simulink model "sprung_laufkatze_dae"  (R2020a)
settings: Solver=ode45  StartTime=0.0  StopTime=20  MaxStep=1e-2  RelTol=1e-5  EnableMultiTasking=on
libraries: simulink x1, simulink_extras x1

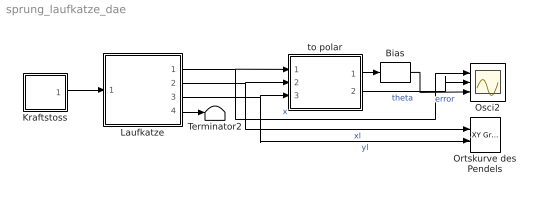
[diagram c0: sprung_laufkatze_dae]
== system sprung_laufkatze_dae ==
  Bias : Bias  Bias=-1
  Kraftstoss : Subsystem  mask(Kraftstoss){Ta=1, Te=10, A=100}
      mask prompts: Ta "Startzeit Te"; Te "Endzeit Ta"; A "Amplitude A"
      mask help: Rechtecksignal, das zur Zeit Te von 0 auf A geht, zur Zeit Ta dann wieder zurück auf 0.
  Laufkatze : Subsystem  mask(Laufkatze){mk=100, ml=1, L=1, g=9.81}
      mask prompts: mk "Laufkatzenmasse"; ml "Lastmasse"; L "Seillaenge"; g "Erdbeschleunigung"
      mask help: DAE-Modell einer Laufkatze als Regelstrecke
  Ortskurve des Pendels : simulink/Sinks/XY Graph  xmin=-1.2  xmax=140  ymin=-1.01  ymax=-0.95  st=-1
  Osci2 : Scope  NumInputPorts=3
  Terminator2 : Terminator
  to polar : Subsystem
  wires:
  Kraftstoss/1(Fext) -> Laufkatze/1(u)
  Laufkatze/1(x) -> to polar/1(x), Osci2/1  "x"
  Laufkatze/2(xl) -> to polar/2(xl), Ortskurve des Pendels/1  "xl"
  Laufkatze/3(yl) -> to polar/3(yl), Ortskurve des Pendels/2  "yl"
  to polar/1(l) -> Bias/1
  Bias/1 -> Osci2/3  "error"
  to polar/2(theta in Grad) -> Osci2/2  "theta"
  Laufkatze/4(lambda) -> Terminator2/1

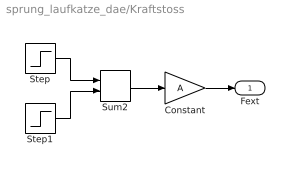
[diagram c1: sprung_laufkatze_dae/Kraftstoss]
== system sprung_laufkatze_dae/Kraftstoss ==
  Constant : Gain  Gain=A  SaturateOnIntegerOverflow=on
  Step : Step  Time=Ta  SampleTime=0
  Step1 : Step  Time=Te  After=-1  SampleTime=0
  Sum2 : Sum  InputSameDT=on  SaturateOnIntegerOverflow=on
  Fext : Outport
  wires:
  Constant/1 -> Fext/1
  Step1/1 -> Sum2/2
  Step/1 -> Sum2/1
  Sum2/1 -> Constant/1

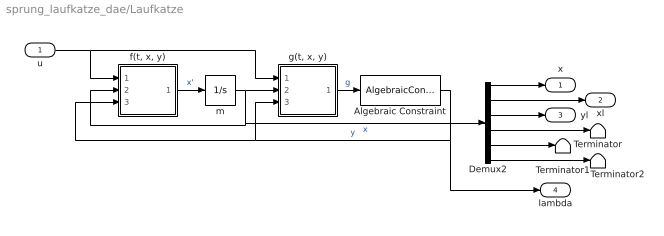
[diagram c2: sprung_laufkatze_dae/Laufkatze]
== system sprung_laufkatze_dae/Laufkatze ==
  u : Inport
  Algebraic Constraint : AlgebraicConstraint
  Demux2 : Demux  Outputs=6
  Terminator : Terminator
  Terminator1 : Terminator
  Terminator2 : Terminator
  "f(t, x, y)" : Subsystem
  "g(t, x, y)" : Subsystem
  m : Integrator  InitialCondition=[0,0,-L,0,0,0]'
  x : Outport
  xl : Outport  Port=2
  yl : Outport  Port=3
  lambda : Outport  Port=4
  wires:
  "g(t, x, y)"/1(g) -> Algebraic Constraint/1  "g"
  Algebraic Constraint/1 -> "g(t, x, y)"/3(y), "f(t, x, y)"/3(y), lambda/1  "y"
  m/1 -> "g(t, x, y)"/2(x), "f(t, x, y)"/2(x), Demux2/1  "x"
  "f(t, x, y)"/1(f) -> m/1  "x'"
  Demux2/1 -> x/1
  Demux2/2 -> xl/1
  Demux2/3 -> yl/1
  Demux2/4 -> Terminator/1
  Demux2/5 -> Terminator1/1
  Demux2/6 -> Terminator2/1
  u/1 -> "g(t, x, y)"/1(u), "f(t, x, y)"/1(u)

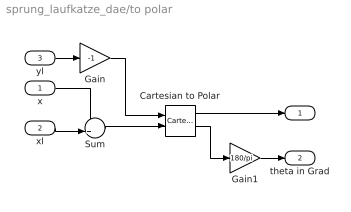
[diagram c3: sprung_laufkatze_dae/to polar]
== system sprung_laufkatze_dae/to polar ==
  x : Inport
  xl : Inport  Port=2
  yl : Inport  Port=3
  Cartesian to Polar : simulink_extras/Transformations/Cartesian to Polar
  Gain : Gain  Gain=-1
  Gain1 : Gain  Gain=180/pi
  Sum : Sum  Inputs=-+|
  l : Outport
  theta in Grad : Outport  Port=2
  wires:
  Cartesian to Polar/2 -> Gain1/1
  Cartesian to Polar/1 -> l/1
  x/1 -> Sum/1
  xl/1 -> Sum/2
  Sum/1 -> Cartesian to Polar/2
  yl/1 -> Gain/1
  Gain/1 -> Cartesian to Polar/1
  Gain1/1 -> theta in Grad/1

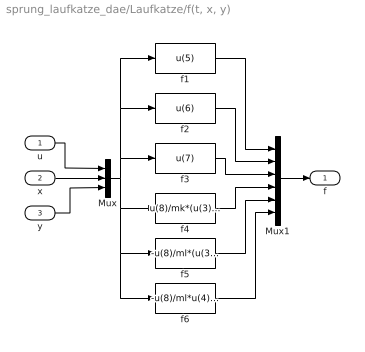
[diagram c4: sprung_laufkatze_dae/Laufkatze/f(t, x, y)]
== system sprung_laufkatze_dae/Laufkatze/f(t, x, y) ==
  u : Inport
  x : Inport  Port=2
  y : Inport  Port=3
  Mux : Mux  Inputs=3
  Mux1 : Mux  Inputs=6
  f1 : Fcn  Expr=u(5)
  f2 : Fcn  Expr=u(6)
  f3 : Fcn  Expr=u(7)
  f4 : Fcn  Expr=u(8)/mk*(u(3)-u(2)) + u(1)/mk
  f5 : Fcn  Expr=-u(8)/ml*(u(3)-u(2))
  f6 : Fcn  Expr=-u(8)/ml*u(4) - g
  f : Outport
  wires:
  u/1 -> Mux/1
  x/1 -> Mux/2
  Mux/1 -> f1/1, f2/1, f3/1, f4/1, f6/1, f5/1
  Mux1/1 -> f/1
  f2/1 -> Mux1/2
  f1/1 -> Mux1/1
  f3/1 -> Mux1/3
  f4/1 -> Mux1/4
  y/1 -> Mux/3
  f5/1 -> Mux1/5
  f6/1 -> Mux1/6

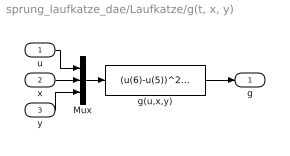
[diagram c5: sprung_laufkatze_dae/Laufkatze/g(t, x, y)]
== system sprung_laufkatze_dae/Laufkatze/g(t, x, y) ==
  u : Inport
  x : Inport  Port=2
  y : Inport  Port=3
  Mux : Mux  Inputs=3
  g(u,x,y) : Fcn  Expr=(u(6)-u(5))^2 + u(7)^2 - u(8)*(1/ml + 1/mk)*(u(3)-u(2))^2 - 1/mk*(u(3)-u(2))*u(1) - u(8)/ml*u(4)^2 - g*u(4)
  g : Outport
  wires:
  u/1 -> Mux/1
  x/1 -> Mux/2
  Mux/1 -> g(u,x,y)/1
  g(u,x,y)/1 -> g/1
  y/1 -> Mux/3
